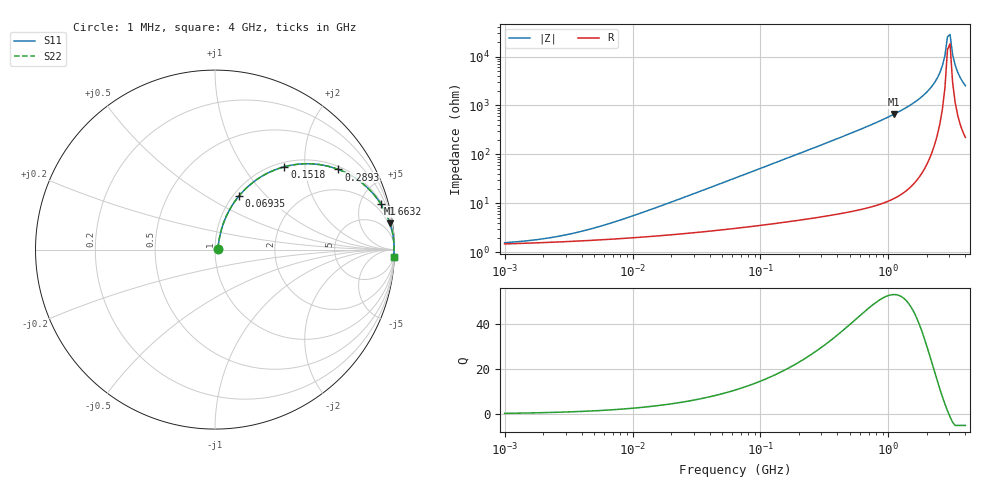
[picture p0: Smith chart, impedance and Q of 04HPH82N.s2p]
# MHz S MA R 50
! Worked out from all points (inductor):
!   181 points, 1 MHz to 4 GHz, reference 50 ohm
!   read as one part in series: L = 82 nH near 12.04 MHz
!   highest Q = 52.8 at 1.101 GHz (marker M1), where L = 95 nH
!   self-resonance near 2.897 GHz
!   S11 on the Smith chart (normalised r, x): 1 MHz: 1.03, +0.01; 69.35 MHz: 1.06, +0.72; 151.8 MHz: 1.08, +1.57; 289.3 MHz: 1.10, +3.01; 663.2 MHz: 1.16, +7.19; 4 GHz: 5, -50
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1  0.01542 18.9  0.9854 -0.3  0.9854 -0.3  0.01542 18.9
2.09018  0.01882 33.7  0.9844 -0.6  0.9844 -0.6  0.01882 33.7
4.1721  0.02703 50.2  0.9829 -1.2  0.9829 -1.2  0.02703 50.2
16.6226  0.08619 70.9  0.9752 -4.8  0.9752 -4.8  0.08619 70.9
63.2456  0.3029 67.1  0.9251 -17.6  0.9251 -17.6  0.3029 67.1
69.351  0.3287 65.8  0.916 -19.1  0.916 -19.1  0.3287 65.8
151.791  0.6026 50.0  0.7674 -37.0  0.7674 -37.0  0.6026 50.0
263.867  0.7943 35.4  0.5792 -52.5  0.5792 -52.5  0.7943 35.4
289.339  0.8201 33.0  0.5446 -55.0  0.5446 -55.0  0.8201 33.0
663.153  0.9581 15.4  0.2664 -73.3  0.2664 -73.3  0.9581 15.4
1051.3  0.9843 9.1  0.1589 -79.8  0.1589 -79.8  0.9843 9.1
1100.88  0.9859 8.6  0.1499 -80.3  0.1499 -80.3  0.9859 8.6
1745.24  0.9955 4.2  0.07252 -84.4  0.07252 -84.4  0.9955 4.2
2301.03  0.9976 1.9  0.03373 -85.0  0.03373 -85.0  0.9976 1.9
2642.15  0.9979 0.9  0.01548 -81.8  0.01548 -81.8  0.9979 0.9
2766.74  0.9979 0.5  0.009545 -77.0  0.009545 -77.0  0.9979 0.5
2897.21  0.9978 0.2  0.003956 -56.6  0.003956 -56.6  0.9978 0.2
3033.83  0.9977 -0.2  0.003533 49.5  0.003533 49.5  0.9977 -0.2
3176.89  0.9975 -0.5  0.009028 73.9  0.009028 73.9  0.9975 -0.5
3326.7  0.9973 -0.8  0.01494 79.2  0.01494 79.2  0.9973 -0.8
3647.85  0.9967 -1.5  0.02701 82.2  0.02701 82.2  0.9967 -1.5
4000  0.9958 -2.2  0.03932 82.7  0.03932 82.7  0.9958 -2.2
